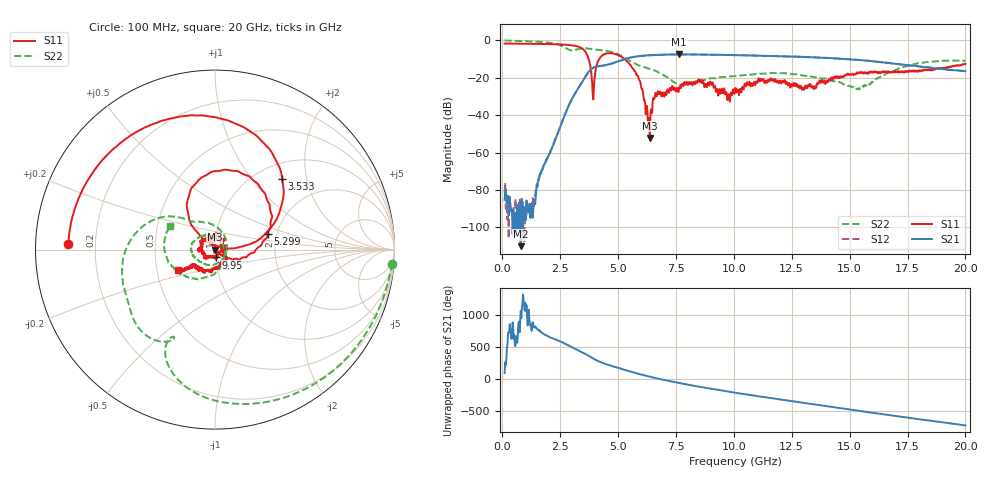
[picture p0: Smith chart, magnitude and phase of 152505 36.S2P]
!  2-Port S-parameters saved by WinCal
! VAR MeasName=S-Parameters (CALIBRATED_DATA) read from VNA (N5230C)
! VAR MeasDate=4/10/2015 9:32:04 AM
! VAR NAME=152505 36
! VAR FILENAME=152505 36.S2P
! VAR DATE=4/10/2015 9:32:04 AM
! VAR PHYS_PORTS=1,2
# Hz S DB R 50
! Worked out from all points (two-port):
!   801 points, 100 MHz to 20 GHz, reference 50 ohm
!   highest |S21| = -7.53 dB at 7.637 GHz (marker M1); lowest = -110.1 dB at 796.5 MHz (marker M2)
!   |S21| within 3 dB of the highest: 5.173 GHz to 15.42 GHz (10.25 GHz wide, 99.5 % of centre)
!   lowest |S11| = -52.2 dB at 6.369 GHz (marker M3), VSWR 1.00, Z = 49.8 - j0.103 ohm
!   |S11| at or under -10 dB: 3.728 GHz to 4.186 GHz (458 MHz wide, 11.6 % of centre); 5.279 GHz to end of sweep
!   |S22| runs from -26.3 to -0.1 dB; largest |S21 - S12| = 0.0048
!   S11 on the Smith chart (normalised r, x): 100 MHz: 0.10, +0.02; 3.533 GHz: 1.29, +1.44; 5.299 GHz: 1.78, +0.35; 9.95 GHz: 1.01, -0.09; 20 GHz: 0.65, -0.16
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1e8  -1.76 177.6  -85.29 89.2  -81.39 -59.3  -0.08 -4.5
7.965e8  -1.81 160.9  -110.06 -21.0  -88.39 110.2  -0.37 -32.3
1.418375e9  -1.90 145.4  -87.60 98.5  -82.75 74.1  -0.69 -57.7
2.53775e9  -2.23 110.8  -44.96 -140.6  -45.06 -141.3  -2.80 -109.2
3.43325e9  -4.27 57.4  -22.52 57.5  -22.52 57.8  -4.34 -124.2
3.53275e9  -5.30 46.4  -20.49 39.6  -20.51 39.8  -4.26 -128.9
3.93075e9  -31.61 100.8  -14.64 -43.6  -14.65 -43.4  -4.86 -146.9
4.32875e9  -7.98 103.1  -13.57 -111.0  -13.57 -111.3  -5.35 -163.3
5.298875e9  -10.27 17.0  -10.04 139.7  -10.02 139.9  -9.39 147.4
5.871e9  -19.54 -29.5  -8.53 79.3  -8.52 79.5  -13.31 131.4
6.3685e9  -52.24 -154.9  -8.01 32.9  -8.02 33.0  -15.32 116.4
6.592375e9  -29.44 102.9  -7.88 14.1  -7.86 14.0  -16.23 105.3
6.741625e9  -27.36 118.9  -7.79 1.7  -7.78 1.5  -17.02 95.7
7.637125e9  -25.53 105.2  -7.53 -66.3  -7.56 -66.2  -23.71 4.7
8.5575e9  -21.41 81.2  -7.64 -127.5  -7.62 -127.5  -21.46 -96.4
9.9505e9  -27.14 -84.2  -7.88 149.1  -7.89 149.0  -19.23 -142.3
1.005e10  -26.72 -93.0  -7.90 143.3  -7.91 143.4  -19.15 -144.9
1.136838e10  -21.67 162.1  -8.35 71.1  -8.29 71.4  -17.79 -173.4
1.338325e10  -24.47 -3.3  -9.09 -34.4  -9.05 -34.2  -19.48 134.3
1.539812e10  -17.68 -116.6  -10.50 -139.4  -10.46 -139.8  -26.25 15.6
1.669162e10  -16.76 -134.2  -12.13 154.0  -12.14 153.2  -17.16 -92.3
2e10  -12.60 -150.2  -16.50 -8.4  -16.46 -8.2  -11.01 151.9
